| IBIS file stm32f7x2_lqfp144.ibs
[IBIS ver] 4.2
[File name] stm32f7x2_lqfp144.ibs
[File Rev] 1.1
[Date]  21-12-2016
[Source] Data Created at STMicroelectronics
[Notes]  File originated from ELDO simulations.
[Disclaimer]  This information is for modeling purpose only and is
   not guaranted.
   The information is subject to change without notice.
[Copyright] Copyright 2017 STMicroelectronics Inc.
|   Component stm32f7x2_lqfp144
[Component] stm32f7x2_lqfp144
[Manufacturer] STMicroelectronics
[Package]
| variable   typ   min   max
R_pkg   0.0   0.0   0.0
L_pkg   0.0H   0.0H   0.0H
C_pkg   0.0F   0.0F   0.0F
[Pin]  signal_name   model_name   R_pin   L_pin   C_pin
1 PE2 io8p_arsudq_ft 187.6E-3 9.4E-9 267.9E-15
2 PE3 io8p_arsudq_ft 182.4E-3 9.1E-9 243.8E-15
3 PE4 io8p_arsudq_ft 177.6E-3 8.7E-9 221.3E-15
4 PE5 io8p_arsudq_ft 173.1E-3 8.4E-9 200.2E-15
5 PE6 io8p_arsudq_ft 168.9E-3 8.1E-9 180.5E-15
6 VBAT power 165.0E-3 7.8E-9 162.3E-15
7 PC13 io8p_arwsudq_ft_v33 161.5E-3 7.6E-9 145.6E-15
8 PC14-OSC32_IN io8p_arwsudq_ft_v33 158.2E-3 7.4E-9 130.3E-15
9 PC15-OSC32_OUT io8p_arwsudq_ft 155.2E-3 7.2E-9 116.4E-15
10 PF0 io8p_arsudq_i2c_ft 152.6E-3 7.0E-9 104.1E-15
11 PF1 io8p_arsudq_i2c_ft 150.3E-3 6.8E-9 93.2E-15
12 PF2 io8p_arsudq_ft 148.2E-3 6.7E-9 83.7E-15
13 PF3 io8p_arwsudq_ft 146.5E-3 6.5E-9 75.7E-15
14 PF4 io8p_arwsudq_ft 145.1E-3 6.4E-9 69.1E-15
15 PF5 io8p_arwsudq_ft 144.1E-3 6.4E-9 64.0E-15
16 VSS gnd 143.3E-3 6.3E-9 60.4E-15
17 VDD power 142.8E-3 6.3E-9 58.2E-15
18 PF6 io8p_arwsudq_ft 142.7E-3 6.3E-9 57.5E-15
19 PF7 io8p_arwsudq_ft 142.7E-3 6.3E-9 57.5E-15
20 PF8 io8p_arwsudq_ft 142.8E-3 6.3E-9 58.2E-15
21 PF9 io8p_arwsudq_ft 143.3E-3 6.3E-9 60.4E-15
22 PF10 io8p_arwsudq_ft 144.1E-3 6.4E-9 64.0E-15
23 PH0-OSC_IN io8p_arsudq_ft 145.1E-3 6.4E-9 69.1E-15
24 PH1-OSC_OUT io8p_arsudq_ft 146.5E-3 6.5E-9 75.7E-15
25 NRST ioreset_ft_v33 148.2E-3 6.7E-9 83.7E-15
26 PC0 io8p_ar3wsudq_ft 150.3E-3 6.8E-9 93.2E-15
27 PC1 io8p_ar3wsudq_ft_v33 152.6E-3 7.0E-9 104.1E-15
28 PC2 io8p_ar3wsudq_ft 155.2E-3 7.2E-9 116.4E-15
29 PC3 io8p_ar3wsudq_ft 158.2E-3 7.4E-9 130.3E-15
30 VDD power 161.5E-3 7.6E-9 145.6E-15
31 VSSA gnd 165.0E-3 7.8E-9 162.3E-15
32 VREF+ power 168.9E-3 8.1E-9 180.5E-15
33 VDDA power 173.1E-3 8.4E-9 200.2E-15
34 PA0-WKUP io8p_ar3wsudq_ft_v33 177.6E-3 8.7E-9 221.3E-15
35 PA1 io8p_ar3wsudq_ft 182.4E-3 9.1E-9 243.8E-15
36 PA2 io8p_ar3wsudq_ft_v33 187.6E-3 9.4E-9 267.9E-15
37 PA3 io8p_ar3wsudq_ft 187.6E-3 9.4E-9 267.9E-15
38 VSS gnd 182.4E-3 9.1E-9 243.8E-15
39 VDD power 177.6E-3 8.7E-9 221.3E-15
40 PA4 io8p_ar3wsudq_ft 173.1E-3 8.4E-9 200.2E-15
41 PA5 io8p_ar3wsudq_ft 168.9E-3 8.1E-9 180.5E-15
42 PA6 io8p_ar3wsudq_ft 165.0E-3 7.8E-9 162.3E-15
43 PA7 io8p_ar3wsudq_ft 161.5E-3 7.6E-9 145.6E-15
44 PC4 io8p_ar3wsudq_ft 158.2E-3 7.4E-9 130.3E-15
45 PC5 io8p_ar3wsudq_ft 155.2E-3 7.2E-9 116.4E-15
46 PB0 io8p_ar3wsudq_ft 152.6E-3 7.0E-9 104.1E-15
47 PB1 io8p_ar3wsudq_ft 150.3E-3 6.8E-9 93.2E-15
48 PB2 io8p_ar3wsudq_ft 148.2E-3 6.7E-9 83.7E-15
49 PF11 io8p_arsudq_ft 146.5E-3 6.5E-9 75.7E-15
50 PF12 io8p_arsudq_ft 145.1E-3 6.4E-9 69.1E-15
51 VSS gnd 144.1E-3 6.4E-9 64.0E-15
52 VDD power 143.3E-3 6.3E-9 60.4E-15
53 PF13 io8p_arsudq_ft 142.8E-3 6.3E-9 58.2E-15
54 PF14 io8p_arsudq_ft 142.7E-3 6.3E-9 57.5E-15
55 PF15 io8p_arsudq_ft 142.7E-3 6.3E-9 57.5E-15
56 PG0 io8p_arsudq_ft 142.8E-3 6.3E-9 58.2E-15
57 PG1 io8p_arsudq_ft 143.3E-3 6.3E-9 60.4E-15
58 PE7 io8p_arsudq_ft 144.1E-3 6.4E-9 64.0E-15
59 PE8 io8p_arsudq_ft 145.1E-3 6.4E-9 69.1E-15
60 PE9 io8p_arsudq_ft 146.5E-3 6.5E-9 75.7E-15
61 VSS gnd 148.2E-3 6.7E-9 83.7E-15
62 VDD power 150.3E-3 6.8E-9 93.2E-15
63 PE10 io8p_arsudq_ft 152.6E-3 7.0E-9 104.1E-15
64 PE11 io8p_arsudq_ft 155.2E-3 7.2E-9 116.4E-15
65 PE12 io8p_arsudq_ft 158.2E-3 7.4E-9 130.3E-15
66 PE13 io8p_arsudq_ft 161.5E-3 7.6E-9 145.6E-15
67 PE14 io8p_arsudq_ft 165.0E-3 7.8E-9 162.3E-15
68 PE15 io8p_ar3wsudq_ft 168.9E-3 8.1E-9 180.5E-15
69 PB10 io8p_arsudq_i2c_ft 173.1E-3 8.4E-9 200.2E-15
70 PB11 io8p_arsudq_i2c_ft 177.6E-3 8.7E-9 221.3E-15
71 VCAP_1 power 182.4E-3 9.1E-9 243.8E-15
72 VDD power 187.6E-3 9.4E-9 267.9E-15
73 PB12 io8usb_id_otg_ft 187.6E-3 9.4E-9 267.9E-15
74 PB13 io8usb_vbus_otg_ft 182.4E-3 9.1E-9 243.8E-15
75 PB14 io8usb_lsfs_otg_ft 177.6E-3 8.7E-9 221.3E-15
76 PB15 io8usb_lsfs_otg_ft 173.1E-3 8.4E-9 200.2E-15
77 PD8 io8p_arsudq_ft 168.9E-3 8.1E-9 180.5E-15
78 PD9 io8p_arsudq_ft 165.0E-3 7.8E-9 162.3E-15
79 PD10 io8p_arsudq_ft 161.5E-3 7.6E-9 145.6E-15
80 PD11 io8p_arsudq_ft 158.2E-3 7.4E-9 130.3E-15
81 PD12 io8p_arsudq_ft 155.2E-3 7.2E-9 116.4E-15
82 PD13 io8p_arsudq_ft 152.6E-3 7.0E-9 104.1E-15
83 VSS gnd 150.3E-3 6.8E-9 93.2E-15
84 VDD power 148.2E-3 6.7E-9 83.7E-15
85 PD14 io8p_arsudq_ft 146.5E-3 6.5E-9 75.7E-15
86 PD15 io8p_arsudq_ft 145.1E-3 6.4E-9 69.1E-15
87 PG2 io8p_arsudq_ft 144.1E-3 6.4E-9 64.0E-15
88 PG3 io8p_arsudq_ft 143.3E-3 6.3E-9 60.4E-15
89 PG4 io8p_arsudq_ft 142.8E-3 6.3E-9 58.2E-15
90 PG5 io8p_arsudq_ft 142.7E-3 6.3E-9 57.5E-15
91 PG6 io8p_arsudq_ft 142.7E-3 6.3E-9 57.5E-15
92 PG7 io8p_arsudq_ft 142.8E-3 6.3E-9 58.2E-15
93 PG8 io8p_arsudq_ft 143.3E-3 6.3E-9 60.4E-15
94 VSS gnd 144.1E-3 6.4E-9 64.0E-15
95 VDDUSB power 145.1E-3 6.4E-9 69.1E-15
96 PC6 io8p_arsudq_ft 146.5E-3 6.5E-9 75.7E-15
97 PC7 io8p_arsudq_ft 148.2E-3 6.7E-9 83.7E-15
98 PC8 io8p_arsudq_ft 150.3E-3 6.8E-9 93.2E-15
99 PC9 io8p_arsudq_i2c_ft 152.6E-3 7.0E-9 104.1E-15
100 PA8 io8p_arsudq_i2c_ft 155.2E-3 7.2E-9 116.4E-15
101 PA9 io8usb_vbus_otg_ft 158.2E-3 7.4E-9 130.3E-15
102 PA10 io8usb_id_otg_ft 161.5E-3 7.6E-9 145.6E-15
103 PA11 io8usb_lsfs_otg_ft 165.0E-3 7.8E-9 162.3E-15
104 PA12 io8usb_lsfs_otg_ft 168.9E-3 8.1E-9 180.5E-15
105 PA13 io8p_arsudq_ft 173.1E-3 8.4E-9 200.2E-15
106 VCAP_2 power 177.6E-3 8.7E-9 221.3E-15
107 VSS gnd 182.4E-3 9.1E-9 243.8E-15
108 VDD power 187.6E-3 9.4E-9 267.9E-15
109 PA14 io8p_arsudq_ft 187.6E-3 9.4E-9 267.9E-15
110 PA15 io8p_arsudq_ft 182.4E-3 9.1E-9 243.8E-15
111 PC10 io8p_arsudq_ft 177.6E-3 8.7E-9 221.3E-15
112 PC11 io8p_arsudq_ft 173.1E-3 8.4E-9 200.2E-15
113 PC12 io8p_arsudq_ft 168.9E-3 8.1E-9 180.5E-15
114 PD0 io8p_arsudq_ft 165.0E-3 7.8E-9 162.3E-15
115 PD1 io8p_arsudq_ft 161.5E-3 7.6E-9 145.6E-15
116 PD2 io8p_arsudq_ft 158.2E-3 7.4E-9 130.3E-15
117 PD3 io8p_arsudq_ft 155.2E-3 7.2E-9 116.4E-15
118 PD4 io8p_arsudq_ft 152.6E-3 7.0E-9 104.1E-15
119 PD5 io8p_arsudq_ft 150.3E-3 6.8E-9 93.2E-15
120 VSS gnd 148.2E-3 6.7E-9 83.7E-15
121 VDDSDMMC power 146.5E-3 6.5E-9 75.7E-15
122 PD6 io8p_arsudq_ft 145.1E-3 6.4E-9 69.1E-15
123 PD7 io8p_arsudq_ft 144.1E-3 6.4E-9 64.0E-15
124 PG9 io8p_arsudq_ft 143.3E-3 6.3E-9 60.4E-15
125 PG10 io8p_arsudq_ft 142.8E-3 6.3E-9 58.2E-15
126 PG11 io8p_arsudq_ft 142.7E-3 6.3E-9 57.5E-15
127 PG12 io8p_arsudq_ft 142.7E-3 6.3E-9 57.5E-15
128 PG13 io8p_arsudq_ft 142.8E-3 6.3E-9 58.2E-15
129 PG14 io8p_arsudq_ft 143.3E-3 6.3E-9 60.4E-15
130 VSS gnd 144.1E-3 6.4E-9 64.0E-15
131 VDD power 145.1E-3 6.4E-9 69.1E-15
132 PG15 io8p_arsudq_ft 146.5E-3 6.5E-9 75.7E-15
133 PB3 io8p_arsudq_ft 148.2E-3 6.7E-9 83.7E-15
134 PB4 io8p_arsudq_ft 150.3E-3 6.8E-9 93.2E-15
135 PB5 io8p_ar3wsudq_ft 152.6E-3 7.0E-9 104.1E-15
136 PB6 io8p_arsudq_i2c_ft 155.2E-3 7.2E-9 116.4E-15
137 PB7 io8p_arsudq_i2c_ft 158.2E-3 7.4E-9 130.3E-15
138 BOOT0 vpp_test_hv 161.5E-3 7.6E-9 145.6E-15
139 PB8 io8p_arsudq_i2c_ft 165.0E-3 7.8E-9 162.3E-15
140 PB9 io8p_arsudq_i2c_ft 168.9E-3 8.1E-9 180.5E-15
141 PE0 io8p_arsudq_ft 173.1E-3 8.4E-9 200.2E-15
142 PE1 io8p_arsudq_ft 177.6E-3 8.7E-9 221.3E-15
143 PDR_ON gnd 182.4E-3 9.1E-9 243.8E-15
144 VDD power 187.6E-3 9.4E-9 267.9E-15
[Diff Pin]   inv_pin   vdiff   tdelay_typ  tdelay_min  tdelay_max
75   76   NA   NA   NA   NA
103   104   NA   NA   NA   NA
[Model Selector] io8p_ar3wsudq_ft
io8p00_ar3wsudq_ft_pd_lv  "SPEED00 1P8V, PD=40kOhm"
io8p00_ar3wsudq_ft_pu_lv  "SPEED00 1P8V, PU=40kOhm"
io8p00_ar3wsudq_ft_lv  "SPEED00 1P8V"
io8p01_ar3wsudq_ft_pd_lv  "SPEED01 1P8V, PD=40kOhm"
io8p01_ar3wsudq_ft_pu_lv  "SPEED01 1P8V, PU=40kOhm"
io8p01_ar3wsudq_ft_lv  "SPEED01 1P8V"
io8p10_ar3wsudq_ft_pd_lv  "SPEED10 1P8V, PD=40kOhm"
io8p10_ar3wsudq_ft_pu_lv  "SPEED10 1P8V, PU=40kOhm"
io8p10_ar3wsudq_ft_lv  "SPEED10 1P8V"
io8p11_ar3wsudq_ft_pd_lv  "SPEED11 1P8V, PD=40kOhm"
io8p11_ar3wsudq_ft_pu_lv  "SPEED11 1P8V, PU=40kOhm"
io8p11_ar3wsudq_ft_lv  "SPEED11 1P8V"
io8p00_ar3wsudq_ft_pd  "SPEED00, PD=40kOhm"
io8p00_ar3wsudq_ft_pu  "SPEED00, PU=40kOhm"
io8p00_ar3wsudq_ft  "SPEED00"
io8p01_ar3wsudq_ft_pd  "SPEED01, PD=40kOhm"
io8p01_ar3wsudq_ft_pu  "SPEED01, PU=40kOhm"
io8p01_ar3wsudq_ft  "SPEED01"
io8p10_ar3wsudq_ft_pd  "SPEED10, PD=40kOhm"
io8p10_ar3wsudq_ft_pu  "SPEED10, PU=40kOhm"
io8p10_ar3wsudq_ft  "SPEED10"
io8p11_ar3wsudq_ft_pd  "SPEED11, PD=40kOhm"
io8p11_ar3wsudq_ft_pu  "SPEED11, PU=40kOhm"
io8p11_ar3wsudq_ft  "SPEED11"
[Model Selector] io8p_ar3wsudq_ft_v33
io8p00_ar3wsudq_ft_v33_pd_lv  "SPEED00 1P8V, PD=40kOhm"
io8p00_ar3wsudq_ft_v33_pu_lv  "SPEED00 1P8V, PU=40kOhm"
io8p00_ar3wsudq_ft_v33_lv  "SPEED00 1P8V"
io8p01_ar3wsudq_ft_v33_pd_lv  "SPEED01 1P8V, PD=40kOhm"
io8p01_ar3wsudq_ft_v33_pu_lv  "SPEED01 1P8V, PU=40kOhm"
io8p01_ar3wsudq_ft_v33_lv  "SPEED01 1P8V"
io8p10_ar3wsudq_ft_v33_pd_lv  "SPEED10 1P8V, PD=40kOhm"
io8p10_ar3wsudq_ft_v33_pu_lv  "SPEED10 1P8V, PU=40kOhm"
io8p10_ar3wsudq_ft_v33_lv  "SPEED10 1P8V"
io8p11_ar3wsudq_ft_v33_pd_lv  "SPEED11 1P8V, PD=40kOhm"
io8p11_ar3wsudq_ft_v33_pu_lv  "SPEED11 1P8V, PU=40kOhm"
io8p11_ar3wsudq_ft_v33_lv  "SPEED11 1P8V"
io8p00_ar3wsudq_ft_v33_pd  "SPEED00, PD=40kOhm"
io8p00_ar3wsudq_ft_v33_pu  "SPEED00, PU=40kOhm"
io8p00_ar3wsudq_ft_v33  "SPEED00"
io8p01_ar3wsudq_ft_v33_pd  "SPEED01, PD=40kOhm"
io8p01_ar3wsudq_ft_v33_pu  "SPEED01, PU=40kOhm"
io8p01_ar3wsudq_ft_v33  "SPEED01"
io8p10_ar3wsudq_ft_v33_pd  "SPEED10, PD=40kOhm"
io8p10_ar3wsudq_ft_v33_pu  "SPEED10, PU=40kOhm"
io8p10_ar3wsudq_ft_v33  "SPEED10"
io8p11_ar3wsudq_ft_v33_pd  "SPEED11, PD=40kOhm"
io8p11_ar3wsudq_ft_v33_pu  "SPEED11, PU=40kOhm"
io8p11_ar3wsudq_ft_v33  "SPEED11"
[Model Selector] io8p_arsudq_ft
io8p00_arsudq_ft_pd_lv  "SPEED00 1P8V, PD=40kOhm"
io8p00_arsudq_ft_pu_lv  "SPEED00 1P8V, PU=40kOhm"
io8p00_arsudq_ft_lv  "SPEED00 1P8V"
io8p01_arsudq_ft_pd_lv  "SPEED01 1P8V, PD=40kOhm"
io8p01_arsudq_ft_pu_lv  "SPEED01 1P8V, PU=40kOhm"
io8p01_arsudq_ft_lv  "SPEED01 1P8V"
io8p10_arsudq_ft_pd_lv  "SPEED10 1P8V, PD=40kOhm"
io8p10_arsudq_ft_pu_lv  "SPEED10 1P8V, PU=40kOhm"
io8p10_arsudq_ft_lv  "SPEED10 1P8V"
io8p11_arsudq_ft_pd_lv  "SPEED11 1P8V, PD=40kOhm"
io8p11_arsudq_ft_pu_lv  "SPEED11 1P8V, PU=40kOhm"
io8p11_arsudq_ft_lv  "SPEED11 1P8V"
io8p00_arsudq_ft_pd  "SPEED00, PD=40kOhm"
io8p00_arsudq_ft_pu  "SPEED00, PU=40kOhm"
io8p00_arsudq_ft  "SPEED00"
io8p01_arsudq_ft_pd  "SPEED01, PD=40kOhm"
io8p01_arsudq_ft_pu  "SPEED01, PU=40kOhm"
io8p01_arsudq_ft  "SPEED01"
io8p10_arsudq_ft_pd  "SPEED10, PD=40kOhm"
io8p10_arsudq_ft_pu  "SPEED10, PU=40kOhm"
io8p10_arsudq_ft  "SPEED10"
io8p11_arsudq_ft_pd  "SPEED11, PD=40kOhm"
io8p11_arsudq_ft_pu  "SPEED11, PU=40kOhm"
io8p11_arsudq_ft  "SPEED11"
[Model Selector] io8p_arsudq_i2c_ft
io8prog_1v8_i2c_pd  "5V Tol GPIO 1.8V range i2c functionality with pull down"
io8prog_1v8_i2c_pu  "5V Tol GPIO 1.8V range i2c functionality with pull up"
io8prog_1v8_i2c  "5V Tol GPIO 1.8V range i2c functionality"
io8prog_3v3_i2c_pd  "5V Tol GPIO 3.3V range i2c functionality with pull down"
io8prog_3v3_i2c_pu  "5V Tol GPIO 3.3V range i2c functionality with pull up"
io8prog_3v3_i2c  "5V Tol GPIO 3.3V range i2c functionality"
io8prog_1v8_pd_00  "5V Tol GPIO 1.8V range with pd speed 00"
io8prog_1v8_pu_00  "5V Tol GPIO 1.8V range with pu speed 00"
io8prog_1v8_00  "5V Tol GPIO 1.8V range speed 00"
io8prog_3v3_pd_00  "5V Tol GPIO 3.3V range with pd speed 00"
io8prog_3v3_pu_00  "5V Tol GPIO 3.3V range with pu speed 00"
io8prog_3v3_00  "5V Tol GPIO 3.3V range speed 00"
io8prog_1v8_pd_01  "5V Tol GPIO 1.8V range with pd speed 01"
io8prog_1v8_pu_01  "5V Tol GPIO 1.8V range with pu speed 01"
io8prog_1v8_01  "5V Tol GPIO 1.8V range speed 01"
io8prog_3v3_pd_01  "5V Tol GPIO 3.3V range with pd speed 01"
io8prog_3v3_pu_01  "5V Tol GPIO 3.3V range with pu speed 01"
io8prog_3v3_01  "5V Tol GPIO 3.3V range speed 01"
io8prog_1v8_pd_10  "5V Tol GPIO 1.8V range with pd speed 10"
io8prog_1v8_pu_10  "5V Tol GPIO 1.8V range with pu speed 10"
io8prog_1v8_10  "5V Tol GPIO 1.8V range speed 10"
io8prog_3v3_pd_10  "5V Tol GPIO 3.3V range with pd speed 10"
io8prog_3v3_pu_10  "5V Tol GPIO 3.3V range with pu speed 10"
io8prog_3v3_10  "5V Tol GPIO 3.3V range speed 10"
io8prog_1v8_pd_11  "5V Tol GPIO 1.8V range with pd speed 11"
io8prog_1v8_pu_11  "5V Tol GPIO 1.8V range with pu speed 11"
io8prog_1v8_11  "5V Tol GPIO 1.8V range speed 11"
io8prog_3v3_pd_11  "5V Tol GPIO 3.3V range with pd speed 11"
io8prog_3v3_pu_11  "5V Tol GPIO 3.3V range with pu speed 11"
io8prog_3v3_11  "5V Tol GPIO 3.3V range speed 11"
[Model Selector] io8p_arwsudq_ft
io8p00_arwsudq_ft_pd_lv  "SPEED00 1P8V, PD=40kOhm"
io8p00_arwsudq_ft_pu_lv  "SPEED00 1P8V, PU=40kOhm"
io8p00_arwsudq_ft_lv  "SPEED00 1P8V"
io8p01_arwsudq_ft_pd_lv  "SPEED01 1P8V, PD=40kOhm"
io8p01_arwsudq_ft_pu_lv  "SPEED01 1P8V, PU=40kOhm"
io8p01_arwsudq_ft_lv  "SPEED01 1P8V"
io8p10_arwsudq_ft_pd_lv  "SPEED10 1P8V, PD=40kOhm"
io8p10_arwsudq_ft_pu_lv  "SPEED10 1P8V, PU=40kOhm"
io8p10_arwsudq_ft_lv  "SPEED10 1P8V"
io8p11_arwsudq_ft_pd_lv  "SPEED11 1P8V, PD=40kOhm"
io8p11_arwsudq_ft_pu_lv  "SPEED11 1P8V, PU=40kOhm"
io8p11_arwsudq_ft_lv  "SPEED11 1P8V"
io8p00_arwsudq_ft_pd  "SPEED00, PD=40kOhm"
io8p00_arwsudq_ft_pu  "SPEED00, PU=40kOhm"
io8p00_arwsudq_ft  "SPEED00"
io8p01_arwsudq_ft_pd  "SPEED01, PD=40kOhm"
io8p01_arwsudq_ft_pu  "SPEED01, PU=40kOhm"
io8p01_arwsudq_ft  "SPEED01"
io8p10_arwsudq_ft_pd  "SPEED10, PD=40kOhm"
io8p10_arwsudq_ft_pu  "SPEED10, PU=40kOhm"
io8p10_arwsudq_ft  "SPEED10"
io8p11_arwsudq_ft_pd  "SPEED11, PD=40kOhm"
io8p11_arwsudq_ft_pu  "SPEED11, PU=40kOhm"
io8p11_arwsudq_ft  "SPEED11"
[Model Selector] io8p_arwsudq_ft_v33
io8p00_arwsudq_ft_v33_pd_lv  "SPEED00 1P8V, PD=40kOhm"
io8p00_arwsudq_ft_v33_pu_lv  "SPEED00 1P8V, PU=40kOhm"
io8p00_arwsudq_ft_v33_lv  "SPEED00 1P8V"
io8p01_arwsudq_ft_v33_pd_lv  "SPEED01 1P8V, PD=40kOhm"
io8p01_arwsudq_ft_v33_pu_lv  "SPEED01 1P8V, PU=40kOhm"
io8p01_arwsudq_ft_v33_lv  "SPEED01 1P8V"
io8p10_arwsudq_ft_v33_pd_lv  "SPEED10 1P8V, PD=40kOhm"
io8p10_arwsudq_ft_v33_pu_lv  "SPEED10 1P8V, PU=40kOhm"
io8p10_arwsudq_ft_v33_lv  "SPEED10 1P8V"
io8p11_arwsudq_ft_v33_pd_lv  "SPEED11 1P8V, PD=40kOhm"
io8p11_arwsudq_ft_v33_pu_lv  "SPEED11 1P8V, PU=40kOhm"
io8p11_arwsudq_ft_v33_lv  "SPEED11 1P8V"
io8p00_arwsudq_ft_v33_pd  "SPEED00, PD=40kOhm"
io8p00_arwsudq_ft_v33_pu  "SPEED00, PU=40kOhm"
io8p00_arwsudq_ft_v33  "SPEED00"
io8p01_arwsudq_ft_v33_pd  "SPEED01, PD=40kOhm"
io8p01_arwsudq_ft_v33_pu  "SPEED01, PU=40kOhm"
io8p01_arwsudq_ft_v33  "SPEED01"
io8p10_arwsudq_ft_v33_pd  "SPEED10, PD=40kOhm"
io8p10_arwsudq_ft_v33_pu  "SPEED10, PU=40kOhm"
io8p10_arwsudq_ft_v33  "SPEED10"
io8p11_arwsudq_ft_v33_pd  "SPEED11, PD=40kOhm"
io8p11_arwsudq_ft_v33_pu  "SPEED11, PU=40kOhm"
io8p11_arwsudq_ft_v33  "SPEED11"
[Model Selector] io8usb_id_otg_ft
io8p00_id_otg_ft_pd_lv  "SPEED00 1P8V, PD=14kOhm"
io8p00_id_otg_ft_pu_lv  "SPEED00 1P8V, PU=14kOhm"
io8p00_id_otg_ft_lv  "SPEED00 1P8V"
io8p01_id_otg_ft_pd_lv  "SPEED01 1P8V, PD=14kOhm"
io8p01_id_otg_ft_pu_lv  "SPEED01 1P8V, PU=14kOhm"
io8p01_id_otg_ft_lv  "SPEED01 1P8V"
io8p10_id_otg_ft_pd_lv  "SPEED10 1P8V, PD=14kOhm"
io8p10_id_otg_ft_pu_lv  "SPEED10 1P8V, PU=14kOhm"
io8p10_id_otg_ft_lv  "SPEED10 1P8V"
io8p11_id_otg_ft_pd_lv  "SPEED11 1P8V, PD=14kOhm"
io8p11_id_otg_ft_pu_lv  "SPEED11 1P8V, PU=14kOhm"
io8p11_id_otg_ft_lv  "SPEED11 1P8V"
io8p00_id_otg_ft_pd  "SPEED00, PD=14kOhm"
io8p00_id_otg_ft_pu  "SPEED00, PU=14kOhm"
io8p00_id_otg_ft  "SPEED00"
io8p01_id_otg_ft_pd  "SPEED01, PD=14kOhm"
io8p01_id_otg_ft_pu  "SPEED01, PU=14kOhm"
io8p01_id_otg_ft  "SPEED01"
io8p10_id_otg_ft_pd  "SPEED10, PD=14kOhm"
io8p10_id_otg_ft_pu  "SPEED10, PU=14kOhm"
io8p10_id_otg_ft  "SPEED10"
io8p11_id_otg_ft_pd  "SPEED11, PD=14kOhm"
io8p11_id_otg_ft_pu  "SPEED11, PU=14kOhm"
io8p11_id_otg_ft  "SPEED11"
[Model Selector] io8usb_lsfs_otg_ft
io8usb_ls_otg_ft_dpdn_pd  "LS USB DP/DN IO + PD=20kOhm"
io8usb_ls_otg_ft_dpdn_pupu2  "LS USB DP/DN IO + PU/PU2=2.2kOhm"
io8usb_ls_otg_ft_dpdn_pu2  "LS USB DP/DN IO + PU2=1.2kOhm"
io8usb_ls_otg_ft_dpdn_pu  "LS USB DP/DN IO + PU=1.2kOhm"
io8usb_ls_otg_ft_dpdn  "LS USB DP/DN IO"
io8usb_fs_otg_ft_dpdn_pd  "HS USB DP/DN IO + PD=20kOhm"
io8usb_fs_otg_ft_dpdn_pupu2  "HS USB DP/DN IO + PU/PU2=2.2kOhm"
io8usb_fs_otg_ft_dpdn_pu2  "HS USB DP/DN IO + PU2=1.2kOhm"
io8usb_fs_otg_ft_dpdn_pu  "HS USB DP/DN IO + PU=1.2kOhm"
io8usb_fs_otg_ft_dpdn  "HS USB DP/DN IO"
io8p00_lsfs_otg_ft_pd_lv  "SPEED00 1P8V, PD=40kOhm"
io8p00_lsfs_otg_ft_pu_lv  "SPEED00 1P8V, PU=40kOhm"
io8p00_lsfs_otg_ft_lv  "SPEED00 1P8V"
io8p01_lsfs_otg_ft_pd_lv  "SPEED01 1P8V, PD=40kOhm"
io8p01_lsfs_otg_ft_pu_lv  "SPEED01 1P8V, PU=40kOhm"
io8p01_lsfs_otg_ft_lv  "SPEED01 1P8V"
io8p10_lsfs_otg_ft_pd_lv  "SPEED10 1P8V, PD=40kOhm"
io8p10_lsfs_otg_ft_pu_lv  "SPEED10 1P8V, PU=40kOhm"
io8p10_lsfs_otg_ft_lv  "SPEED10 1P8V"
io8p11_lsfs_otg_ft_pd_lv  "SPEED11 1P8V, PD=40kOhm"
io8p11_lsfs_otg_ft_pu_lv  "SPEED11 1P8V, PU=40kOhm"
io8p11_lsfs_otg_ft_lv  "SPEED11 1P8V"
io8p00_lsfs_otg_ft_pd  "SPEED00, PD=40kOhm"
io8p00_lsfs_otg_ft_pu  "SPEED00, PU=40kOhm"
io8p00_lsfs_otg_ft  "SPEED00"
io8p01_lsfs_otg_ft_pd  "SPEED01, PD=40kOhm"
io8p01_lsfs_otg_ft_pu  "SPEED01, PU=40kOhm"
io8p01_lsfs_otg_ft  "SPEED01"
io8p10_lsfs_otg_ft_pd  "SPEED10, PD=40kOhm"
io8p10_lsfs_otg_ft_pu  "SPEED10, PU=40kOhm"
io8p10_lsfs_otg_ft  "SPEED10"
io8p11_lsfs_otg_ft_pd  "SPEED11, PD=40kOhm"
io8p11_lsfs_otg_ft_pu  "SPEED11, PU=40kOhm"
io8p11_lsfs_otg_ft  "SPEED11"
[Model Selector] io8usb_vbus_otg_ft
io8psenb_vbus_otg_ft  "VBUS PULSE, SENSE VB"
io8psenab_vbus_otg_ft  "VBUS PULSE, SENSE VA and VB"
io8psena_vbus_otg_ft  "VBUS PULSE, SENSE VA"
io8psen_vbus_otg_ft  "VBUS PULSE"
io8p00_vbus_otg_ft_pd_lv  "SPEED00 1P8V, PD=40kOhm"
io8p00_vbus_otg_ft_pu_lv  "SPEED00 1P8V, PU=40kOhm"
io8p00_vbus_otg_ft_lv  "SPEED00 1P8V"
io8p01_vbus_otg_ft_pd_lv  "SPEED01 1P8V, PD=40kOhm"
io8p01_vbus_otg_ft_pu_lv  "SPEED01 1P8V, PU=40kOhm"
io8p01_vbus_otg_ft_lv  "SPEED01 1P8V"
io8p10_vbus_otg_ft_pd_lv  "SPEED10 1P8V, PD=40kOhm"
io8p10_vbus_otg_ft_pu_lv  "SPEED10 1P8V, PU=40kOhm"
io8p10_vbus_otg_ft_lv  "SPEED10 1P8V"
io8p11_vbus_otg_ft_pd_lv  "SPEED11 1P8V, PD=40kOhm"
io8p11_vbus_otg_ft_pu_lv  "SPEED11 1P8V, PU=40kOhm"
io8p11_vbus_otg_ft_lv  "SPEED11 1P8V"
io8p00_vbus_otg_ft_pd  "SPEED00, PD=40kOhm"
io8p00_vbus_otg_ft_pu  "SPEED00, PU=40kOhm"
io8p00_vbus_otg_ft  "SPEED00"
io8p01_vbus_otg_ft_pd  "SPEED01, PD=40kOhm"
io8p01_vbus_otg_ft_pu  "SPEED01, PU=40kOhm"
io8p01_vbus_otg_ft  "SPEED01"
io8p10_vbus_otg_ft_pd  "SPEED10, PD=40kOhm"
io8p10_vbus_otg_ft_pu  "SPEED10, PU=40kOhm"
io8p10_vbus_otg_ft  "SPEED10"
io8p11_vbus_otg_ft_pd  "SPEED11, PD=40kOhm"
io8p11_vbus_otg_ft_pu  "SPEED11, PU=40kOhm"
io8p11_vbus_otg_ft  "SPEED11"
[Model Selector] ioreset_ft_v33
ioreset_ft_v33_pu_lv  "IORESET 1P8V + PU=40kOhm"
ioreset_ft_v33_nopu_lv  "IORESET 1P8V"
ioreset_ft_v33_pu  "IORESET + PU=40kOhm"
ioreset_ft_v33_nopu  "IORESET"
[Model Selector] vpp_test_hv
vpp_test_hv_2p4  "Input Buffer 1P8V"
vpp_test_hv_3p3  "Input Buffer"
| Models and submodels in the file (242): io8p00_ar3wsudq_ft_pd_lv (I/O), io8p00_ar3wsudq_ft_pu_lv (I/O), io8p00_ar3wsudq_ft_lv (I/O), io8p01_ar3wsudq_ft_pd_lv (I/O), io8p01_ar3wsudq_ft_pu_lv (I/O), io8p01_ar3wsudq_ft_lv (I/O), io8p10_ar3wsudq_ft_pd_lv (I/O), io8p10_ar3wsudq_ft_pu_lv (I/O), io8p10_ar3wsudq_ft_lv (I/O), io8p11_ar3wsudq_ft_pd_lv (I/O), io8p11_ar3wsudq_ft_pu_lv (I/O), io8p11_ar3wsudq_ft_lv (I/O), io8p00_ar3wsudq_ft_pd (I/O), io8p00_ar3wsudq_ft_pu (I/O), io8p00_ar3wsudq_ft (I/O), io8p01_ar3wsudq_ft_pd (I/O), io8p01_ar3wsudq_ft_pu (I/O), io8p01_ar3wsudq_ft (I/O), io8p10_ar3wsudq_ft_pd (I/O), io8p10_ar3wsudq_ft_pu (I/O), io8p10_ar3wsudq_ft (I/O), io8p11_ar3wsudq_ft_pd (I/O), io8p11_ar3wsudq_ft_pu (I/O), io8p11_ar3wsudq_ft (I/O), io8p00_ar3wsudq_ft_v33_pd_lv (I/O), io8p00_ar3wsudq_ft_v33_pu_lv (I/O), io8p00_ar3wsudq_ft_v33_lv (I/O), io8p01_ar3wsudq_ft_v33_pd_lv (I/O), io8p01_ar3wsudq_ft_v33_pu_lv (I/O), io8p01_ar3wsudq_ft_v33_lv (I/O), io8p10_ar3wsudq_ft_v33_pd_lv (I/O), io8p10_ar3wsudq_ft_v33_pu_lv (I/O), io8p10_ar3wsudq_ft_v33_lv (I/O), io8p11_ar3wsudq_ft_v33_pd_lv (I/O), io8p11_ar3wsudq_ft_v33_pu_lv (I/O), io8p11_ar3wsudq_ft_v33_lv (I/O), io8p00_ar3wsudq_ft_v33_pd (I/O), io8p00_ar3wsudq_ft_v33_pu (I/O), io8p00_ar3wsudq_ft_v33 (I/O), io8p01_ar3wsudq_ft_v33_pd (I/O), io8p01_ar3wsudq_ft_v33_pu (I/O), io8p01_ar3wsudq_ft_v33 (I/O), io8p10_ar3wsudq_ft_v33_pd (I/O), io8p10_ar3wsudq_ft_v33_pu (I/O), io8p10_ar3wsudq_ft_v33 (I/O), io8p11_ar3wsudq_ft_v33_pd (I/O), io8p11_ar3wsudq_ft_v33_pu (I/O), io8p11_ar3wsudq_ft_v33 (I/O), io8p00_arsudq_ft_pd_lv (I/O), io8p00_arsudq_ft_pu_lv (I/O), io8p00_arsudq_ft_lv (I/O), io8p01_arsudq_ft_pd_lv (I/O), io8p01_arsudq_ft_pu_lv (I/O), io8p01_arsudq_ft_lv (I/O), io8p10_arsudq_ft_pd_lv (I/O), io8p10_arsudq_ft_pu_lv (I/O), io8p10_arsudq_ft_lv (I/O), io8p11_arsudq_ft_pd_lv (I/O), io8p11_arsudq_ft_pu_lv (I/O), io8p11_arsudq_ft_lv (I/O), io8p00_arsudq_ft_pd (I/O), io8p00_arsudq_ft_pu (I/O), io8p00_arsudq_ft (I/O), io8p01_arsudq_ft_pd (I/O), io8p01_arsudq_ft_pu (I/O), io8p01_arsudq_ft (I/O), io8p10_arsudq_ft_pd (I/O), io8p10_arsudq_ft_pu (I/O), io8p10_arsudq_ft (I/O), io8p11_arsudq_ft_pd (I/O), io8p11_arsudq_ft_pu (I/O), io8p11_arsudq_ft (I/O), io8prog_1v8_i2c_pd (I/O), io8prog_1v8_i2c_pu (I/O), io8prog_1v8_i2c (I/O), io8prog_3v3_i2c_pd (I/O), io8prog_3v3_i2c_pu (I/O), io8prog_3v3_i2c (I/O), io8prog_1v8_pd_00 (I/O), io8prog_1v8_pu_00 (I/O)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
